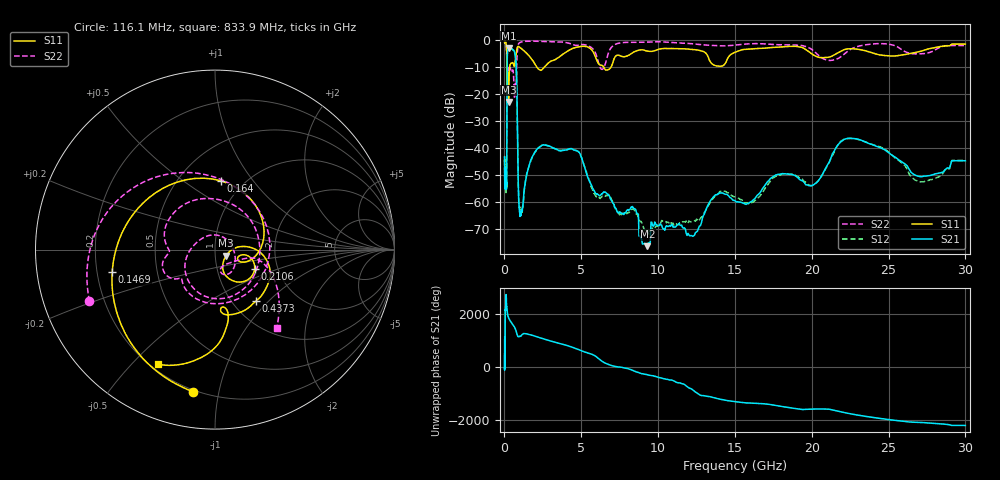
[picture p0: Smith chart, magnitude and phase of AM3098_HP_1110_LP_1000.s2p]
! Date/Time: Thu, Feb 28, 2019 8:46 AM
! Network Analyzer: Agilent Technologies E8364B Rev: A.07.50.67
! Sweep from 0.010 to 30.000 GHz, 1601 Points, Sweep Type: LOG
! Power Supply: 5.022 V, 0.002 A
# Hz S DB R 50
!freq MagS11 AngS11 MagS21 AngS21 MagS12 AngS12 MagS22 AngS22
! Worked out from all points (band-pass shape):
!   1601 points, 10 MHz to 30 GHz, reference 50 ohm
!   highest |S21| = -3.03 dB at 293 MHz (marker M1); lowest = -76.3 dB at 9.302 GHz (marker M2)
!   |S21| within 3 dB of the highest: 183.7 MHz to 707.9 MHz (524.2 MHz wide, 118 % of centre)
!   lowest |S11| = -23.0 dB at 266.5 MHz (marker M3), VSWR 1.15, Z = 56.5 - j3.87 ohm
!   |S11| at or under -10 dB: 169.7 MHz to 342.9 MHz (173.2 MHz wide, 67.6 % of centre); 2.094 GHz to 2.619 GHz (525.3 MHz wide, 22.3 % of centre); 6.455 GHz to 6.953 GHz (497.8 MHz wide, 7.43 % of centre)
!   |S22| runs from -21.8 to -0.5 dB; largest |S21 - S12| = 0.011
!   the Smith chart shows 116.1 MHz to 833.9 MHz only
!   S11 on the Smith chart (normalised r, x): 116.1 MHz: 0.19, -0.84; 146.9 MHz: 0.26, -0.10; 164 MHz: 0.79, +0.71; 210.6 MHz: 1.52, -0.36; 437.3 MHz: 1.28, -0.84; 833.9 MHz: 0.23, -0.60
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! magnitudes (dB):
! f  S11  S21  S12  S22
! 10 MHz  -0.4  -43.3  -44.3  -0.6
! 38.04 MHz  -0.3  -51.1  -50.5  -0.7
! 116.1 MHz  -1.9  -53.3  -54.0  -2.4
! 144.7 MHz  -4.3  -50.6  -52.5  -5.5
! 146.9 MHz  -4.6  -48.1  -49.6  -6.1
! 164 MHz  -8.3  -19.7  -19.7  -10.4
! 210.6 MHz  -12.2  -4.0  -4.0  -10.4
! 266.5 MHz  -23.0  -3.1  -3.1  -11.9
! 293 MHz  -16.0  -3.0  -3.0  -11.5
! 437.3 MHz  -8.7  -3.2  -3.2  -11.6
! 550.5 MHz  -8.6  -3.8  -3.8  -11.3
! 739.5 MHz  -6.1  -7.7  -7.7  -19.8
! 833.9 MHz  -2.9  -27.9  -27.9  -5.1
! 917.1 MHz  -2.5  -57.2  -57.4  -1.5
! 1.024 GHz  -3.0  -64.8  -62.3  -1.0
! 2.084 GHz  -9.9  -40.7  -41.0  -0.6
! 4.71 GHz  -2.8  -41.1  -41.0  -2.1
! 7.926 GHz  -6.1  -63.6  -64.0  -1.0
! 9.302 GHz  -4.2  -76.3  -70.3  -0.9
! 20 GHz  -5.2  -54.0  -54.0  -3.6
! 22.56 GHz  -3.3  -36.5  -36.5  -3.5
! 30 GHz  -1.6  -44.8  -44.6  -2.2
